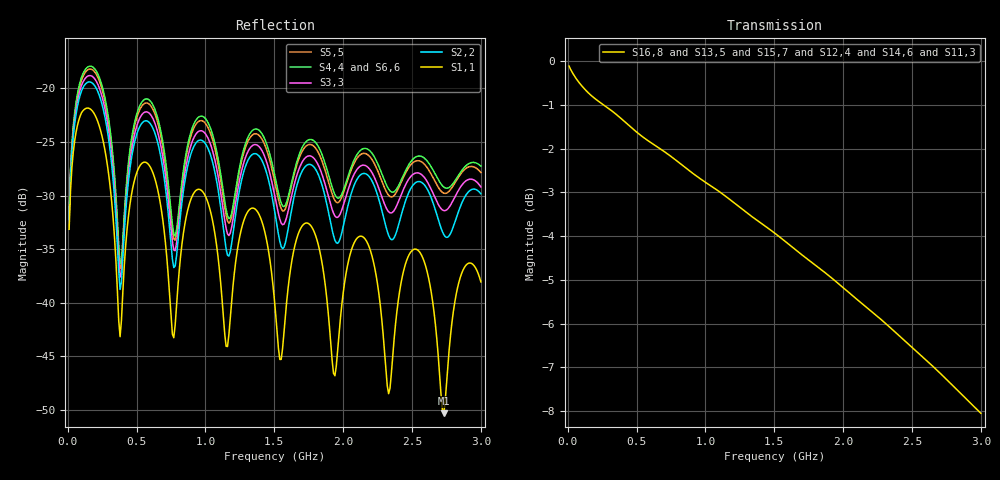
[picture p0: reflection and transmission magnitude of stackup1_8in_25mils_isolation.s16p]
! Touchstone file from project
# GHZ S RI R 50.000000
! Modal data exported
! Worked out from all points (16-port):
!   300 points, 10 MHz to 3 GHz, reference 50 ohm
!   strongest paths, dB at 10 MHz, 760 MHz, 1.51 GHz, 2.26 GHz, 3 GHz:
!     S16,8: -0.1, -2.2, -3.9, -5.9, -8.1
!     S13,5: -0.1, -2.2, -4.0, -6.0, -8.2
!     S15,7: -0.1, -2.2, -4.0, -6.0, -8.2
!     S12,4: -0.1, -2.2, -4.0, -6.0, -8.2
!     S14,6: -0.1, -2.2, -4.0, -6.0, -8.3
!     S11,3: -0.1, -2.2, -4.0, -6.0, -8.3
!   lowest |S11| = -50.3 dB at 2.73 GHz (marker M1), VSWR 1.01, Z = 50.3 - j0.116 ohm
!   |S11| at or under -10 dB: start of sweep to end of sweep
